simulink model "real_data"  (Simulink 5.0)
settings: Solver=ode45  StartTime=0.0  StopTime=0.399  MaxStep=T_s
libraries: simulink x1

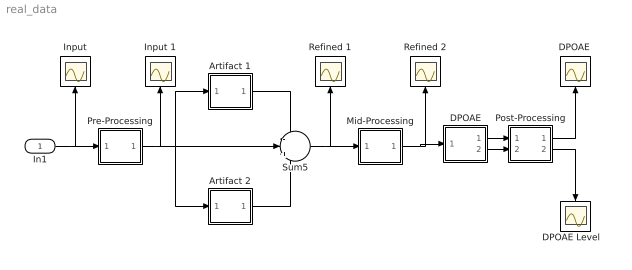
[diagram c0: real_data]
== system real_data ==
  In1 : Inport
  Artifact 1 : Subsystem
  Artifact 2 : Subsystem
  DPOAE : Subsystem
  "DPOAE Level   " : Scope
  "DPOAE " : Scope
  Input : Scope
  Input 1 : Scope
  Mid-Processing : Subsystem
  Post-Processing : Subsystem
  Pre-Processing : Subsystem
  Refined 1 : Scope
  Refined 2 : Scope
  Sum5 : Sum  Inputs=-|+|-
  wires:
  Pre-Processing/1(Out1) -> Input 1/1, Sum5/2, Artifact 1/1(In1), Artifact 2/1(In1)
  Sum5/1 -> Mid-Processing/1(In1), Refined 1/1
  Mid-Processing/1(Out1) -> DPOAE/1(In1), Refined 2/1
  Artifact 1/1(Out1) -> Sum5/1
  Artifact 2/1(Out1) -> Sum5/3
  In1/1 -> Pre-Processing/1(In1), Input/1
  Post-Processing/1(Out1) -> "DPOAE "/1
  Post-Processing/2(Out2) -> "DPOAE Level   "/1
  DPOAE/1(Out1) -> Post-Processing/1(In1)
  DPOAE/2(Out2) -> Post-Processing/2(In2)

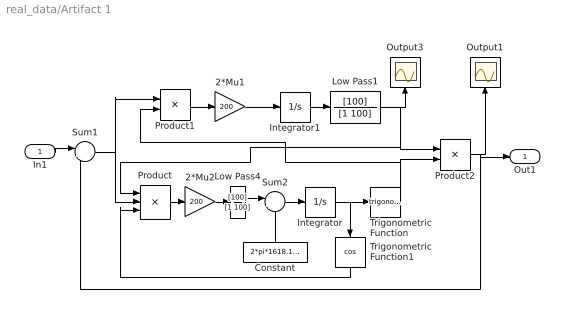
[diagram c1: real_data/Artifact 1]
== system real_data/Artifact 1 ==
  In1 : Inport
  2*Mu1 : Gain  Gain=200
  2*Mu2 : Gain  Gain=200
  Constant : Constant  Orientation=up  Value=2*pi*1618.16394
  Integrator : Integrator
  Integrator1 : Integrator
  Low Pass1 : TransferFcn  Numerator=[100]  Denominator=[1 100]
  Low Pass4 : TransferFcn  Numerator=[100]  Denominator=[1 100]
  Output1 : Scope
  Output3 : Scope
  Product : Product  Inputs=3
  Product1 : Product
  Product2 : Product
  Sum1 : Sum  Inputs=|+-
  Sum2 : Sum  Inputs=|++
  Trigonometric Function : Trigonometry
  Trigonometric Function1 : Trigonometry  Orientation=down  Operator=cos
  Out1 : Outport
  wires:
  Product1/1 -> 2*Mu1/1
  2*Mu1/1 -> Integrator1/1
  Sum2/1 -> Integrator/1
  Constant/1 -> Sum2/2
  Trigonometric Function/1 -> Product2/2, Product1/2
  Integrator/1 -> Trigonometric Function/1, Trigonometric Function1/1
  Product2/1 -> Output1/1, Sum1/2, Out1/1
  Integrator1/1 -> Low Pass1/1
  Low Pass1/1 -> Output3/1, Product2/1, Product/1
  2*Mu2/1 -> Low Pass4/1
  Low Pass4/1 -> Sum2/1
  Trigonometric Function1/1 -> Product/3
  Sum1/1 -> Product1/1, Product/2
  Product/1 -> 2*Mu2/1
  In1/1 -> Sum1/1

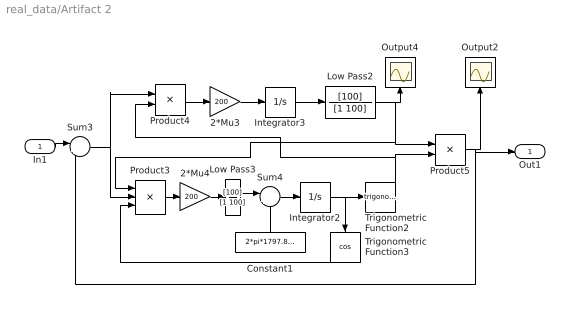
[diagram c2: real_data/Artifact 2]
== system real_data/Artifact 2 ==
  In1 : Inport
  2*Mu3 : Gain  Gain=200
  2*Mu4 : Gain  Gain=200
  Constant1 : Constant  Orientation=up  Value=2*pi*1797.851440
  Integrator2 : Integrator
  Integrator3 : Integrator
  Low Pass2 : TransferFcn  Numerator=[100]  Denominator=[1 100]
  Low Pass3 : TransferFcn  Numerator=[100]  Denominator=[1 100]
  Output2 : Scope
  Output4 : Scope
  Product3 : Product  Inputs=3
  Product4 : Product
  Product5 : Product
  Sum3 : Sum  Inputs=|+-
  Sum4 : Sum  Inputs=|++
  Trigonometric Function2 : Trigonometry
  Trigonometric Function3 : Trigonometry  Orientation=down  Operator=cos
  Out1 : Outport
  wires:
  Product4/1 -> 2*Mu3/1
  2*Mu3/1 -> Integrator3/1
  Sum4/1 -> Integrator2/1
  Constant1/1 -> Sum4/2
  Trigonometric Function2/1 -> Product5/2, Product4/2
  Integrator2/1 -> Trigonometric Function2/1, Trigonometric Function3/1
  Product5/1 -> Sum3/2, Output2/1, Out1/1
  Integrator3/1 -> Low Pass2/1
  Low Pass2/1 -> Output4/1, Product5/1, Product3/1
  2*Mu4/1 -> Low Pass3/1
  Low Pass3/1 -> Sum4/1
  Product3/1 -> 2*Mu4/1
  Trigonometric Function3/1 -> Product3/3
  Sum3/1 -> Product4/1, Product3/2
  In1/1 -> Sum3/1

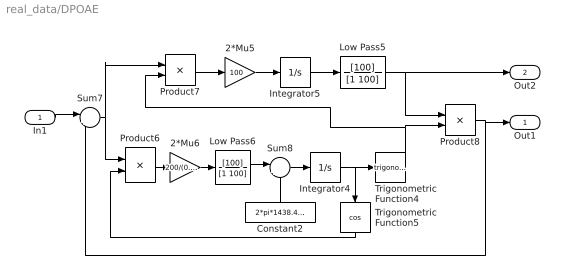
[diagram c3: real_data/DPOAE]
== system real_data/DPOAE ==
  In1 : Inport
  2*Mu5 : Gain  Gain=100
  2*Mu6 : Gain  Gain=200/(0.005)
  Constant2 : Constant  Orientation=up  Value=2*pi*1438.47644
  Integrator4 : Integrator
  Integrator5 : Integrator
  Low Pass5 : TransferFcn  Numerator=[100]  Denominator=[1 100]
  Low Pass6 : TransferFcn  Numerator=[100]  Denominator=[1 100]
  Product6 : Product
  Product7 : Product
  Product8 : Product
  Sum7 : Sum  Inputs=|+-
  Sum8 : Sum  Inputs=|++
  Trigonometric Function4 : Trigonometry
  Trigonometric Function5 : Trigonometry  Orientation=down  Operator=cos
  Out1 : Outport
  Out2 : Outport  Port=2
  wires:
  Product7/1 -> 2*Mu5/1
  Product6/1 -> 2*Mu6/1
  2*Mu5/1 -> Integrator5/1
  Trigonometric Function4/1 -> Product8/2, Product7/2
  Integrator4/1 -> Trigonometric Function4/1, Trigonometric Function5/1
  Trigonometric Function5/1 -> Product6/2
  Product8/1 -> Out1/1, Sum7/2
  Constant2/1 -> Sum8/2
  Sum7/1 -> Product7/1, Product6/1
  Integrator5/1 -> Low Pass5/1
  2*Mu6/1 -> Low Pass6/1
  Low Pass5/1 -> Product8/1, Out2/1
  Low Pass6/1 -> Sum8/1
  Sum8/1 -> Integrator4/1
  In1/1 -> Sum7/1

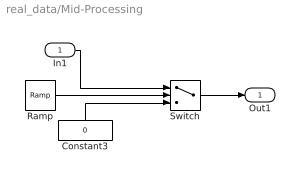
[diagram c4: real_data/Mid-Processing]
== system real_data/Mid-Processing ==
  In1 : Inport
  Constant3 : Constant  Orientation=up  Value=0
  Ramp : simulink/Sources/Ramp  slope=1  start=0  X0=0
  Switch : Switch  Threshold=.1
  Out1 : Outport
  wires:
  Constant3/1 -> Switch/3
  Ramp/1 -> Switch/2
  In1/1 -> Switch/1
  Switch/1 -> Out1/1

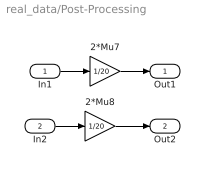
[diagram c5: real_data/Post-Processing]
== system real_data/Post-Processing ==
  In1 : Inport
  In2 : Inport  Port=2
  2*Mu7 : Gain  Gain=1/20
  2*Mu8 : Gain  Gain=1/20
  Out1 : Outport
  Out2 : Outport  Port=2
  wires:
  In1/1 -> 2*Mu7/1
  2*Mu7/1 -> Out1/1
  In2/1 -> 2*Mu8/1
  2*Mu8/1 -> Out2/1

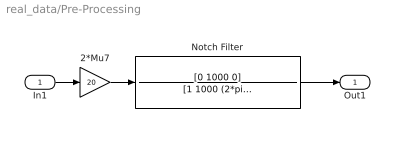
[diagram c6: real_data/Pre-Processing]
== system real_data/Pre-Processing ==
  In1 : Inport
  2*Mu7 : Gain  Gain=20
  Notch Filter : TransferFcn  Numerator=[0 1000 0]  Denominator=[1 1000 (2*pi*1438.47644)^2]
  Out1 : Outport
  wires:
  2*Mu7/1 -> Notch Filter/1
  In1/1 -> 2*Mu7/1
  Notch Filter/1 -> Out1/1
